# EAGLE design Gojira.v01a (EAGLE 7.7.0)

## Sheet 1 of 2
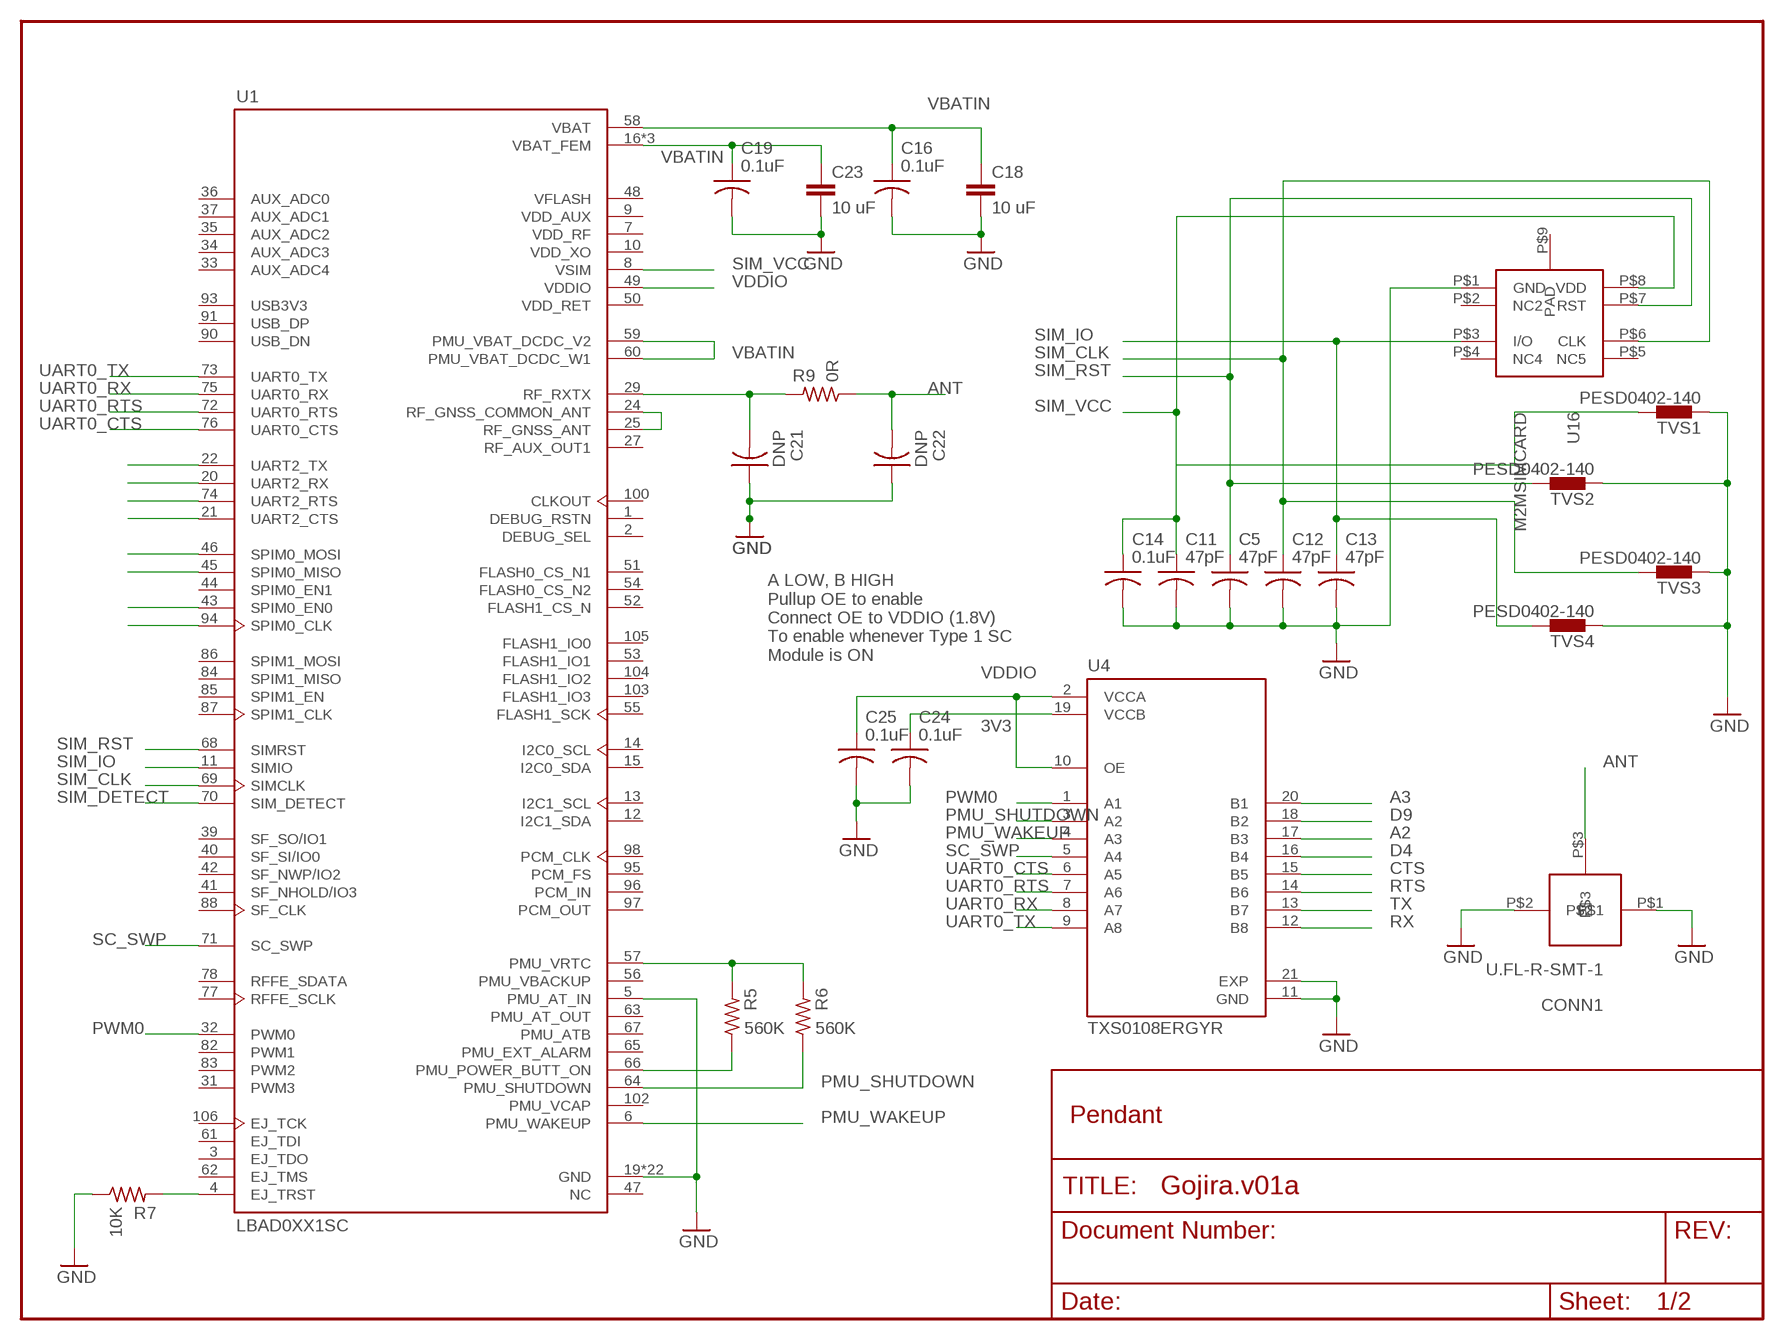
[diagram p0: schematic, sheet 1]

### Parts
C5  47pF  C-US  [C0402_B]
C11  47pF  C-US  [C0402_B]
C12  47pF  C-US  [C0402_B]
C13  47pF  C-US  [C0402_B]
C14  0.1uF  C-US  [C0402_B]
C16  0.1uF  C-US  [C0402_B]
C18  10 uF  CAP0603-CAP  [0603-CAP]
C19  0.1uF  C-US  [C0402_B]
C21  DNP  C-US  [C0402_B]
C22  DNP  C-US  [C0402_B]
C23  10 uF  CAP0603-CAP  [0603-CAP]
C24  0.1uF  C-US  [C0402_B]
C25  0.1uF  C-US  [C0402_B]
CONN1  U.FL-R-SMT-1  [U.FL-R-SMT-1]
R5  560K  R-US_  [R0402_B]
R6  560K  R-US_  [R0402_B]
R7  10K  R-US_  [R0402_B]
R9  0R  R-US_  [R0402_B]
TVS1  PESD0402-140  BLM15H  [0402]
TVS2  PESD0402-140  BLM15H  [0402]
TVS3  PESD0402-140  BLM15H  [0402]
TVS4  PESD0402-140  BLM15H  [0402]
U1  LBAD0XX1SC  [XCVR_LBAD0XX1SC]
U4  TXS0108ERGYR  [IC_TXS0108ERGYR]
U16  M2MSIMCARD  [M2MSIMCARD]

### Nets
3V3: C24.1 U4.19(VCCB) ; also sheet 2
A2: U4.17(B3) ; also sheet 2
A3: U4.20(B1) ; also sheet 2
ANT: C22.2 CONN1.P$3 R9.1
CTS: U4.15(B5) ; also sheet 2
D4: U4.16(B4) ; also sheet 2
D9: U4.18(B2) ; also sheet 2
GND: C5.2 C11.2 C12.2 C13.2 C14.2 C16.2 C18.2 C19.2 C21.1 C22.1 C23.2 C24.2 C25.2 CONN1.P$1 CONN1.P$2 R7.1 TVS1.1 TVS2.1 TVS3.1 TVS4.1 U1.5(PMU_AT_IN) U1.19(GND) U1.23(GND) U1.26(GND) U1.28(GND) U1.30(GND) U1.38(GND) U1.79(GND) U1.80(GND) U1.81(GND) U1.89(GND) U1.92(GND) U1.99(GND) U1.101(GND) U1.107(GND) U1.108(GND) U1.109(GND) U1.110(GND) U1.111(GND) U1.112(GND) U1.113(GND) U1.114(GND) U1.115(GND) U4.11(GND) U4.21(EXP) U16.P$1(GND) ; also sheet 2
N$3: R5.2 R6.2 U1.57(PMU_VRTC)
N$5: R5.1 U1.66(PMU_POWER_BUTT_ON)
N$9: U1.24(RF_GNSS_COMMON_ANT) U1.25(RF_GNSS_ANT)
N$10: R7.2 U1.4(EJ_TRST)
N$13: U1.20(UART2_RX)
N$14: U1.22(UART2_TX)
N$16: U1.21(UART2_CTS)
N$17: U1.74(UART2_RTS)
N$18: U1.43(SPIM0_EN0)
N$19: U1.45(SPIM0_MISO)
N$20: U1.46(SPIM0_MOSI)
N$21: U1.94(SPIM0_CLK)
PMU_SHUTDOWN: R6.1 U1.64(PMU_SHUTDOWN) U4.3(A2)
PMU_WAKEUP: U1.6(PMU_WAKEUP) U4.4(A3)
PWM0: U1.32(PWM0) U4.1(A1)
RF_OUT: C21.2 R9.2 U1.29(RF_RXTX)
RTS: U4.14(B6) ; also sheet 2
RX: U4.12(B8) ; also sheet 2
SC_SWP: U1.71(SC_SWP) U4.5(A4)
SIM_CLK: C12.1 TVS3.2 U1.69(SIMCLK) U16.P$6(CLK)
SIM_DETECT: U1.70(SIM_DETECT)
SIM_IO: C13.1 TVS4.2 U1.11(SIMIO) U16.P$3(I/O)
SIM_RST: C5.1 TVS2.2 U1.68(SIMRST) U16.P$7(RST)
SIM_VCC: C11.1 C14.1 TVS1.2 U1.8(VSIM) U16.P$8(VDD)
TX: U4.13(B7) ; also sheet 2
UART0_CTS: U1.76(UART0_CTS) U4.6(A5)
UART0_RTS: U1.72(UART0_RTS) U4.7(A6)
UART0_RX: U1.75(UART0_RX) U4.8(A7)
UART0_TX: U1.73(UART0_TX) U4.9(A8)
VBATIN: C16.1 C18.1 C19.1 C23.1 U1.16(VBAT_FEM) U1.17(VBAT_FEM) U1.18(VBAT_FEM) U1.58(VBAT) U1.59(PMU_VBAT_DCDC_V2) U1.60(PMU_VBAT_DCDC_W1) ; also sheet 2
VDDIO: C25.1 U1.49(VDDIO) U4.2(VCCA) U4.10(OE)
Unconnected: U1.1(DEBUG_RSTN) U1.2(DEBUG_SEL) U1.3(EJ_TDO) U1.7(VDD_RF) U1.9(VDD_AUX) U1.10(VDD_XO) U1.12(I2C1_SDA) U1.13(I2C1_SCL) U1.14(I2C0_SCL) U1.15(I2C0_SDA) U1.27(RF_AUX_OUT1) U1.31(PWM3) U1.33(AUX_ADC4) U1.34(AUX_ADC3) U1.35(AUX_ADC2) U1.36(AUX_ADC0) U1.37(AUX_ADC1) U1.39(SF_SO/IO1) U1.40(SF_SI/IO0) U1.41(SF_NHOLD/IO3) U1.42(SF_NWP/IO2) U1.44(SPIM0_EN1) U1.47(NC) U1.48(VFLASH) U1.50(VDD_RET) U1.51(FLASH0_CS_N1) U1.52(FLASH1_CS_N) U1.53(FLASH1_IO1) U1.54(FLASH0_CS_N2) U1.55(FLASH1_SCK) U1.56(PMU_VBACKUP) U1.61(EJ_TDI) U1.62(EJ_TMS) U1.63(PMU_AT_OUT) U1.65(PMU_EXT_ALARM) U1.67(PMU_ATB) U1.77(RFFE_SCLK) U1.78(RFFE_SDATA) U1.82(PWM1) U1.83(PWM2) U1.84(SPIM1_MISO) U1.85(SPIM1_EN) U1.86(SPIM1_MOSI) U1.87(SPIM1_CLK) U1.88(SF_CLK) U1.90(USB_DN) U1.91(USB_DP) U1.93(USB3V3) U1.95(PCM_FS) U1.96(PCM_IN) U1.97(PCM_OUT) U1.98(PCM_CLK) U1.100(CLKOUT) U1.102(PMU_VCAP) U1.103(FLASH1_IO3) U1.104(FLASH1_IO2) U1.105(FLASH1_IO0) U1.106(EJ_TCK) U16.P$2(NC2) U16.P$4(NC4) U16.P$5(NC5)

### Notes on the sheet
- A LOW, B HIGH
  Pullup OE to enable
  Connect OE to VDDIO (1.8V)
  To enable whenever Type 1 SC
  Module is ON
- Pendant

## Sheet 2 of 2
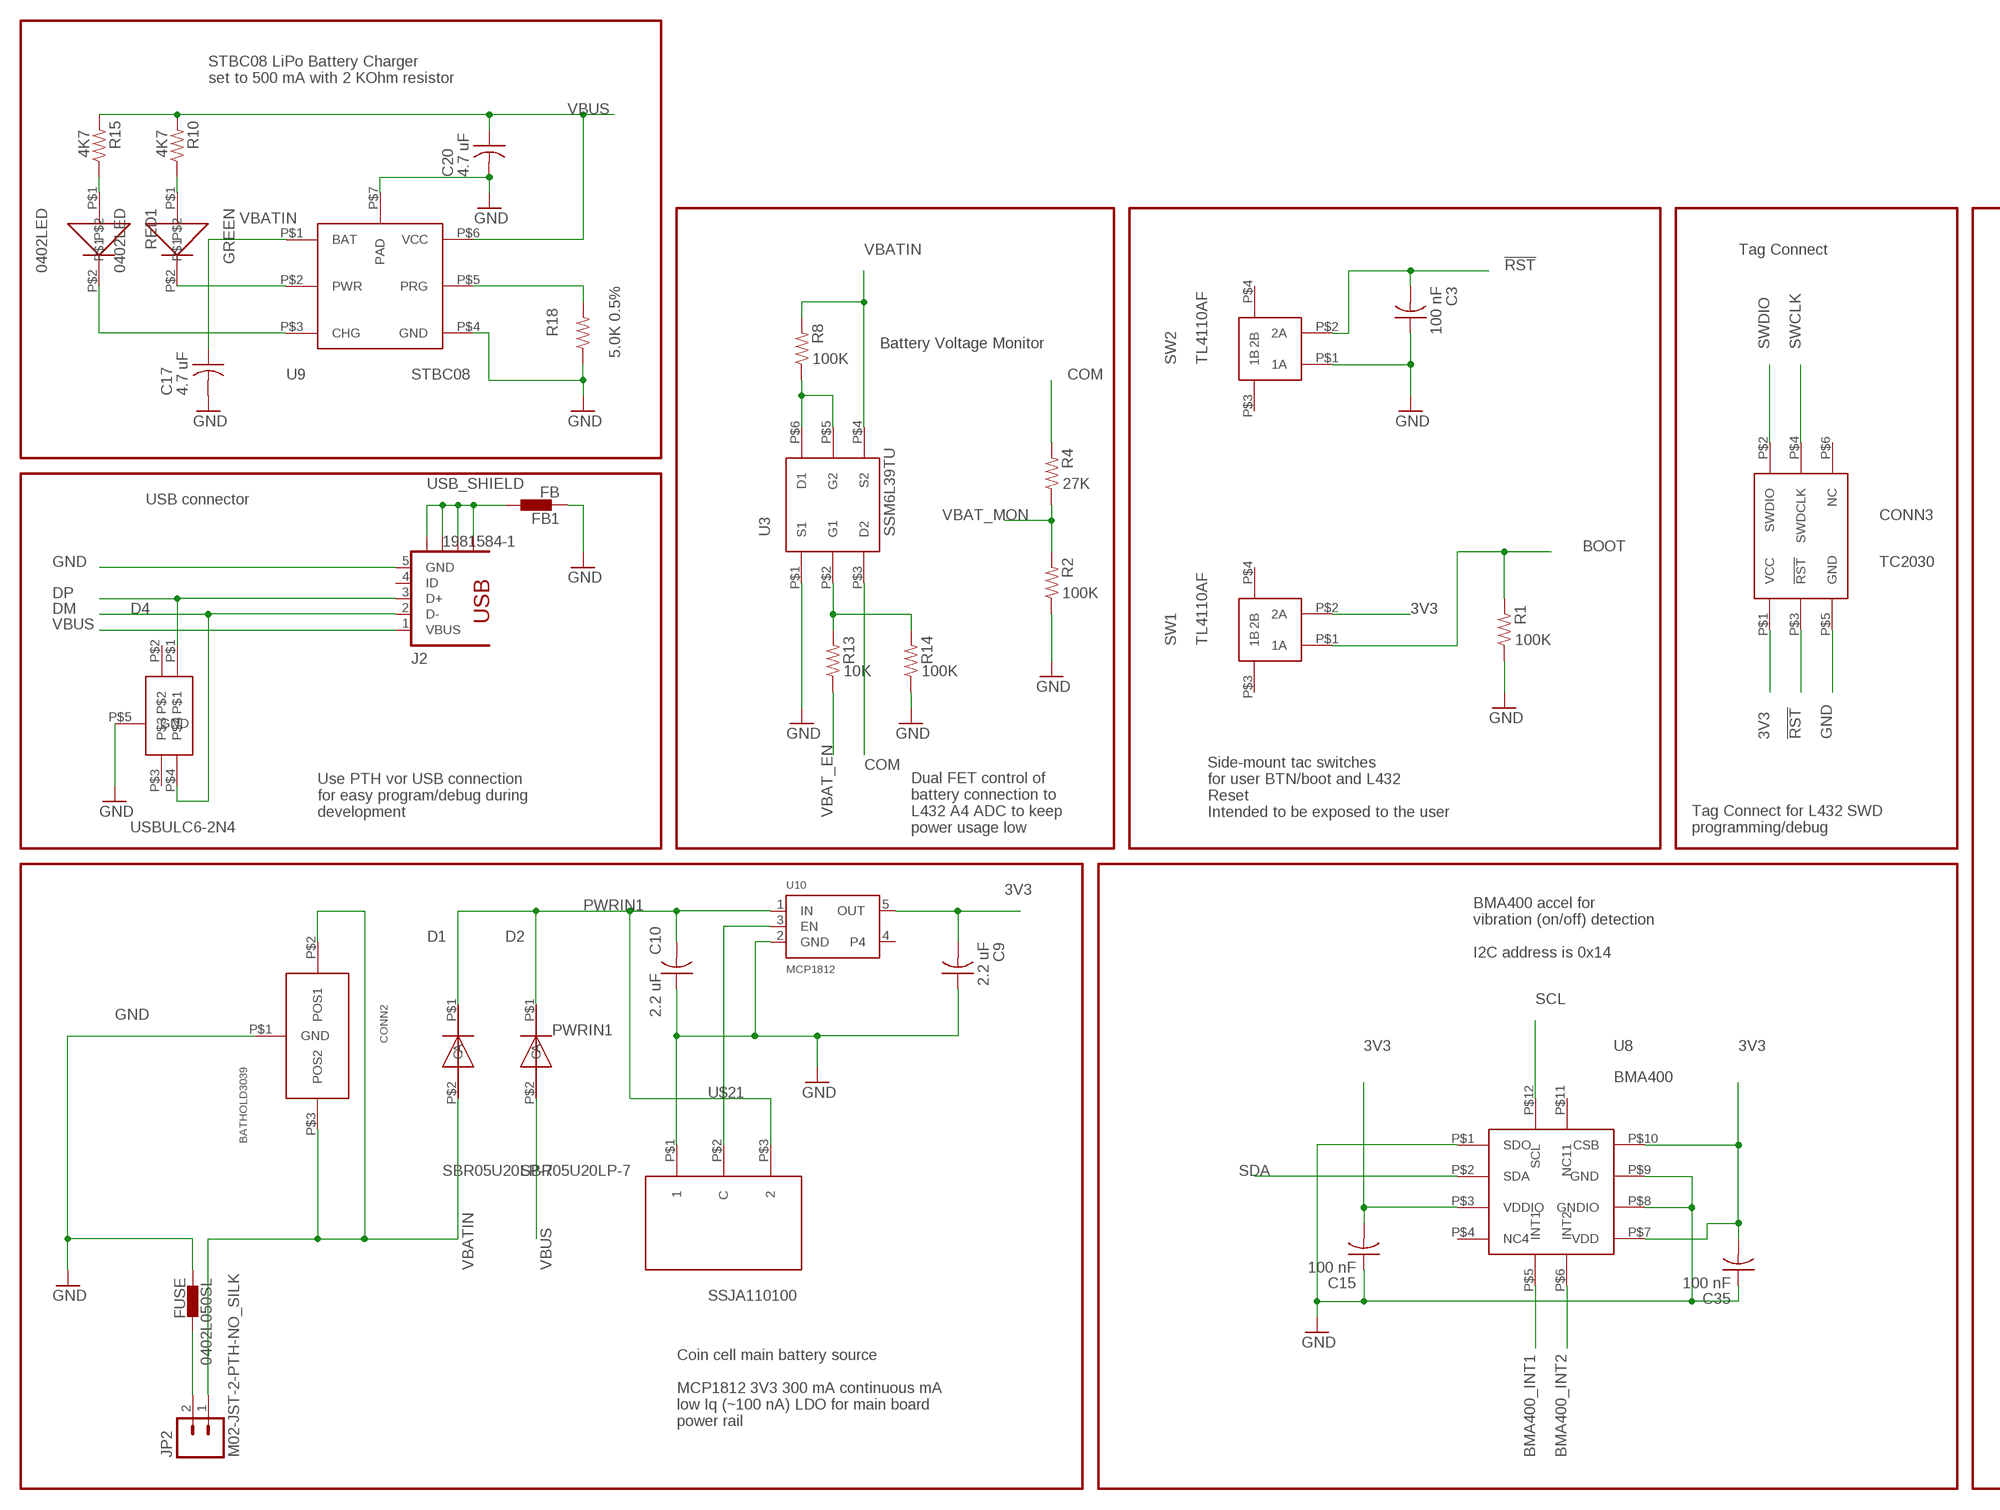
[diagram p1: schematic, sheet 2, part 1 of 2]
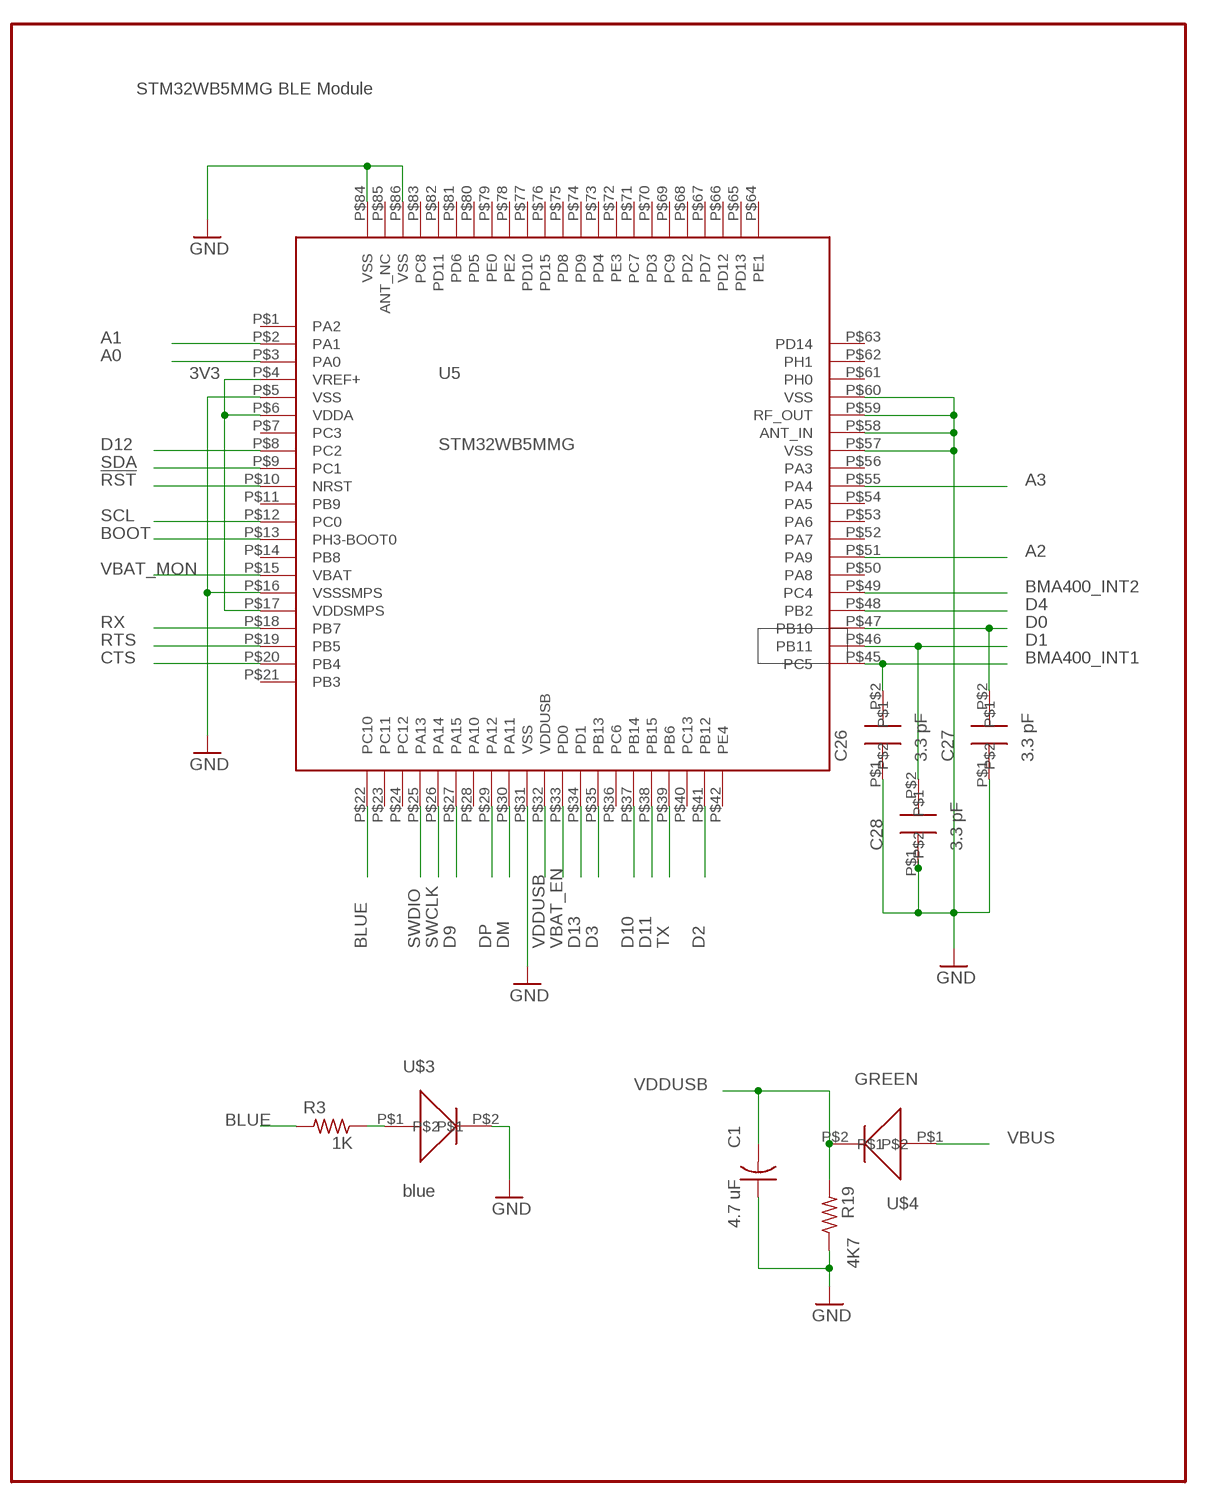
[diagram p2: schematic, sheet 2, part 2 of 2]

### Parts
0402L050SL  FUSE  BLM15H  [0402]
C1  4.7 uF  C-US  [C0402_B]
C3  100 nF  C-US  [C0402_B]
C9  2.2 uF  C-US  [C0402_B]
C10  2.2 uF  C-US  [C0402_B]
C15  100 nF  C-US  [C0402_B]
C17  4.7 uF  C-US  [C0402_B]
C20  4.7 uF  C-US  [C0402_B]
C26  3.3 pF  201CAP  [0201CAP]
C27  3.3 pF  201CAP  [0201CAP]
C28  3.3 pF  201CAP  [0201CAP]
C35  100 nF  C-US  [C0402_B]
CONN2  BATHOLD3039  [BATHOLD3039]
CONN3  TC2030  [TC2030]
D1  SBR05U20LP-7  CDSQR4148-HF  [CDSQR4148-HF]
D2  SBR05U20LP-7  CDSQR4148-HF  [CDSQR4148-HF]
D4  USBULC6-2N4  [USBULC6-2N4]
FB1  FB  BLM15H  [0402]
GREEN  0402LED  [0402LED]
J2  1981584-1  [1981584-1]
JP2  M02-JST-2-PTH-NO_SILK  [JST-2-PTH-NS]
R1  100K  R-US_  [R0402_B]
R2  100K  R-US_  [R0402_B]
R3  1K  R-US_  [R0402_B]
R4  27K  R-US_  [R0402_B]
R8  100K  R-US_  [R0402_B]
R10  4K7  R-US_  [R0402_B]
R13  10K  R-US_  [R0402_B]
R14  100K  R-US_  [R0402_B]
R15  4K7  R-US_  [R0402_B]
R18  5.0K 0.5%  R-US_  [R0402_B]
R19  4K7  R-US_  [R0402_B]
RED1  0402LED  [0402LED]
SW1  TL4110AF  [TL4110AF]
SW2  TL4110AF  [TL4110AF]
U3  SSM6L39TU  [SSM6L39TU]
U5  STM32WB5MMG  [STM32WB5MMG]
U8  BMA400  [BMA400]
U9  STBC08  [STBC08]
U10  MCP1812  VREG_SOT23-5  [SOT23-5]
U$3  blue  0402LED  [0402LED]
U$4  GREEN  0402LED  [0402LED]
U$21  SSJA110100  [SSAJ110100]

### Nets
3V3: C9.2 C15.2 C35.2 CONN3.P$1(VCC) SW1.P$2(2A) U5.P$4(VREF+) U5.P$6(VDDA) U5.P$17(VDDSMPS) U8.P$3(VDDIO) U8.P$7(VDD) U8.P$10(CSB) U10.5(OUT) ; also sheet 1
!RST: C3.2 CONN3.P$3(!RST) SW2.P$2(2A) U5.P$10(NRST)
A0: U5.P$3(PA0)
A1: U5.P$2(PA1)
A2: U5.P$51(PA9) ; also sheet 1
A3: U5.P$55(PA4) ; also sheet 1
BLUE: R3.2 U5.P$22(PC10)
BMA400_INT1: C26.P$2 U5.P$45(PC5) U8.P$5(INT1)
BMA400_INT2: U5.P$49(PC4) U8.P$6(INT2)
BOOT: R1.2 SW1.P$1(1A) U5.P$13(PH3-BOOT0)
COM: R4.2 U3.P$3(D2)
CTS: U5.P$20(PB4) ; also sheet 1
D0: C27.P$2 U5.P$47(PB10)
D1: C28.P$2 U5.P$46(PB11)
D2: U5.P$41(PB12)
D3: U5.P$35(PB13)
D4: U5.P$48(PB2) ; also sheet 1
D9: U5.P$27(PA15) ; also sheet 1
D10: U5.P$37(PB14)
D11: U5.P$38(PB15)
D12: U5.P$8(PC2)
D13: U5.P$34(PD1)
DM: D4.P$4 J2.2(D-) U5.P$30(PA11)
DP: D4.P$1 J2.3(D+) U5.P$29(PA12)
GND: 0402L050SL.1 C1.1 C3.1 C9.1 C10.1 C15.1 C17.2 C20.2 C26.P$1 C27.P$1 C28.P$1 C35.1 CONN2.P$1(GND) CONN3.P$5(GND) D4.P$5(GND) FB1.1 J2.5(GND) R1.1 R2.1 R14.1 R18.1 R19.1 SW2.P$1(1A) U3.P$1(S1) U5.P$5(VSS) U5.P$16(VSSSMPS) U5.P$31(VSS) U5.P$57(VSS) U5.P$58(ANT_IN) U5.P$59(RF_OUT) U5.P$60(VSS) U5.P$84(VSS) U5.P$86(VSS) U8.P$1(SDO) U8.P$8(GNDIO) U8.P$9(GND) U9.P$4(GND) U9.P$7(PAD) U10.2(GND) U$3.P$2 U$21.P$1 ; also sheet 1
N$1: R15.1 RED1.P$1
N$4: 0402L050SL.2 JP2.2
N$7: R13.2 R14.2 U3.P$2(G1)
N$11: R3.1 U$3.P$1
N$15: R8.1 U3.P$5(G2) U3.P$6(D1)
N$22: RED1.P$2 U9.P$3(CHG)
N$23: GREEN.P$2 U9.P$2(PWR)
N$24: GREEN.P$1 R10.1
N$25: U10.3(EN) U$21.P$2(C)
N$27: R18.2 U9.P$5(PRG)
PWRIN1: C10.2 D1.P$1(C) D2.P$1(C) U10.1(IN) U$21.P$3
RTS: U5.P$19(PB5) ; also sheet 1
RX: U5.P$18(PB7) ; also sheet 1
SCL: U5.P$12(PC0) U8.P$12(SCL)
SDA: U5.P$9(PC1) U8.P$2(SDA)
SWCLK: CONN3.P$4(SWDCLK) U5.P$26(PA14)
SWDIO: CONN3.P$2(SWDIO) U5.P$25(PA13)
TX: U5.P$39(PB6) ; also sheet 1
USB_SHIELD: FB1.2 J2.S1 J2.S2 J2.S3 J2.S4
VBAT_EN: R13.1 U5.P$33(PD0)
VBAT_MON: R2.2 R4.1 U5.P$15(VBAT)
VBATIN: C17.1 CONN2.P$2(POS1) CONN2.P$3(POS2) D1.P$2(A) JP2.1 R8.2 U3.P$4(S2) U9.P$1(BAT) ; also sheet 1
VBUS: C20.1 D2.P$2(A) J2.1(VBUS) R10.2 R15.2 U9.P$6(VCC) U$4.P$1
VDDUSB: C1.2 R19.2 U5.P$32(VDDUSB) U$4.P$2
Unconnected: CONN3.P$6(NC) D4.P$2 D4.P$3 J2.4(ID) SW1.P$3(1B) SW1.P$4(2B) SW2.P$3(1B) SW2.P$4(2B) U5.P$1(PA2) U5.P$7(PC3) U5.P$11(PB9) U5.P$14(PB8) U5.P$21(PB3) U5.P$23(PC11) U5.P$24(PC12) U5.P$28(PA10) U5.P$36(PC6) U5.P$40(PC13) U5.P$42(PE4) U5.P$50(PA8) U5.P$52(PA7) U5.P$53(PA6) U5.P$54(PA5) U5.P$56(PA3) U5.P$61(PH0) U5.P$62(PH1) U5.P$63(PD14) U5.P$64(PE1) U5.P$65(PD13) U5.P$66(PD12) U5.P$67(PD7) U5.P$68(PD2) U5.P$69(PC9) U5.P$70(PD3) U5.P$71(PC7) U5.P$72(PE3) U5.P$73(PD4) U5.P$74(PD9) U5.P$75(PD8) U5.P$76(PD15) U5.P$77(PD10) U5.P$78(PE2) U5.P$79(PE0) U5.P$80(PD5) U5.P$81(PD6) U5.P$82(PD11) U5.P$83(PC8) U5.P$85(ANT_NC) U8.P$4(NC4) U8.P$11(NC11) U10.4

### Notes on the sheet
- STBC08 LiPo Battery Charger
  set to 500 mA with 2 KOhm resistor
- Tag Connect
- STM32WB5MMG BLE Module
- Battery Voltage Monitor
- USB connector
- Use PTH vor USB connection
  for easy program/debug during
  development
- Side-mount tac switches
  for user BTN/boot and L432 
  Reset
  Intended to be exposed to the user
- Dual FET control of
  battery connection to
  L432 A4 ADC to keep
  power usage low
- Tag Connect for L432 SWD 
  programming/debug
- BMA400 accel for
  vibration (on/off) detection
  
  I2C address is 0x14
- Coin cell main battery source
  
  MCP1812 3V3 300 mA continuous mA
  low Iq (~100 nA) LDO for main board 
  power rail

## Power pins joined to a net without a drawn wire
PAD: U16.P$9(PAD)

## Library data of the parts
0402L050SL FB1 TVS1-TVS4 = STM32L433SARA.AssetTracker.v01:BLM15H: EMIFIL (R) Chip Ferrite Bead for GHz Noise
C1 C3 C5 C9-C17 C19-C22 C24 C25 C35 = Spark:C-US: Capacitor
C18 C23 = SparkFun-Capacitors:CAP: Capacitor
C26-C28 = Kris:201CAP: 0201 capacitor for high-density applications (STM32WB5MMG)
CONN1 = Kris:U.FL-R-SMT-1: U.FL-R-SMT-1
CONN2 = Kris:BATHOLD3039: 2450 battery holder file:///C:/Users/kris/AppData/Local/Temp/3039.PDF
CONN3 = Kris:TC2030: TC2030 SWD pogo pin contact pad
D1 D2 = Kris:CDSQR4148-HF: ComChip's CDSQR4148-HF high speed 150 mA Io diode
D4 = Kris:USBULC6-2N4: ST TVS diode ESD Protection USBULC6-2N4
GREEN RED1 U$3 U$4 = Kris:0402LED: 0402led
J2 = con-usb:1981584-1: Receptacle, micro-USB, type A/B Tyco Electronics; MF: Hirose; MPN: ZX62-AB-5PA(11)
JP2 = SparkFun-Connectors:M02: Standard 2-pin 0.1" header. Use with
R1-R10 R13-R15 R18 R19 = Spark:R-US_: 0402 Resistor
SW1 SW2 = Kris:TL4110AF: TL4110AF side-mounted tac switch
U1 = LBAD0XX1SC:LBAD0XX1SC: LTE CAT M1 Module Check prices; AVAILABILITY: Bad; DESCRIPTION: Bluetooth Development Tools (802.15.1); MF: Murata Power Solutions; MP: LBAD0XX1SC; PACKAGE: None; PRICE: None
U3 = Kris:SSM6L39TU: SSM6L39TU Dual Mosfet https://www.mouser.com/datasheet/2/408/SSM6L39TU_datasheet_en_20140301-771389.pdf
U4 = TXS0108ERGYR:TXS0108ERGYR: 8-bit bidirectional voltage-level shifter for open-drain and push-pull application 20-VQFN -40 to 85; DESCRIPTION: 8-bit bidirectional voltage-level shifter for open-drain and push-pull application 20-VQFN -40 to 85; DIGI-KEY_PART_NUMBER: 296-24806-1-ND; MF: Texas Instruments; MP: TXS0108ERGYR; PACKAGE: VQFN-20 Texas Instruments; PURCHASE-URL: https://pricing.snapeda.com/search/part/TXS0108ERGYR/?ref=eda
U5 = Kris:STM32WB5MMG: STM32WB5MMG BLE Module
U8 = Kris:BMA400: BMA400 https://ae-bst.resource.bosch.com/media/_tech/media/datasheets/BST-BMA400-DS000-02.pdf
U9 = Kris:STBC08: STBC08
U10 = ModernDevice:VREG_SOT23-5: SOT23-5 Fixed Voltage Regulators To better organise some of the SOT23-5 fixed voltage regulators in this library, this new part was created. Part Current Out V Out V In V Dropout Digikey Part No. ADP121 150mA 3.3V 3.4-5.5V 0.09V @ 150mA ADP121-AUJZ33R7CT-ND ADP121 150mA 3.0V 3.1-5.5V 0.09V @ 150mA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
U16 = Kris:M2MSIMCARD: M2M Sim Card
U$21 = Kris:SSJA110100: ALPS SSJA110100 SPDT slide switch with lugs

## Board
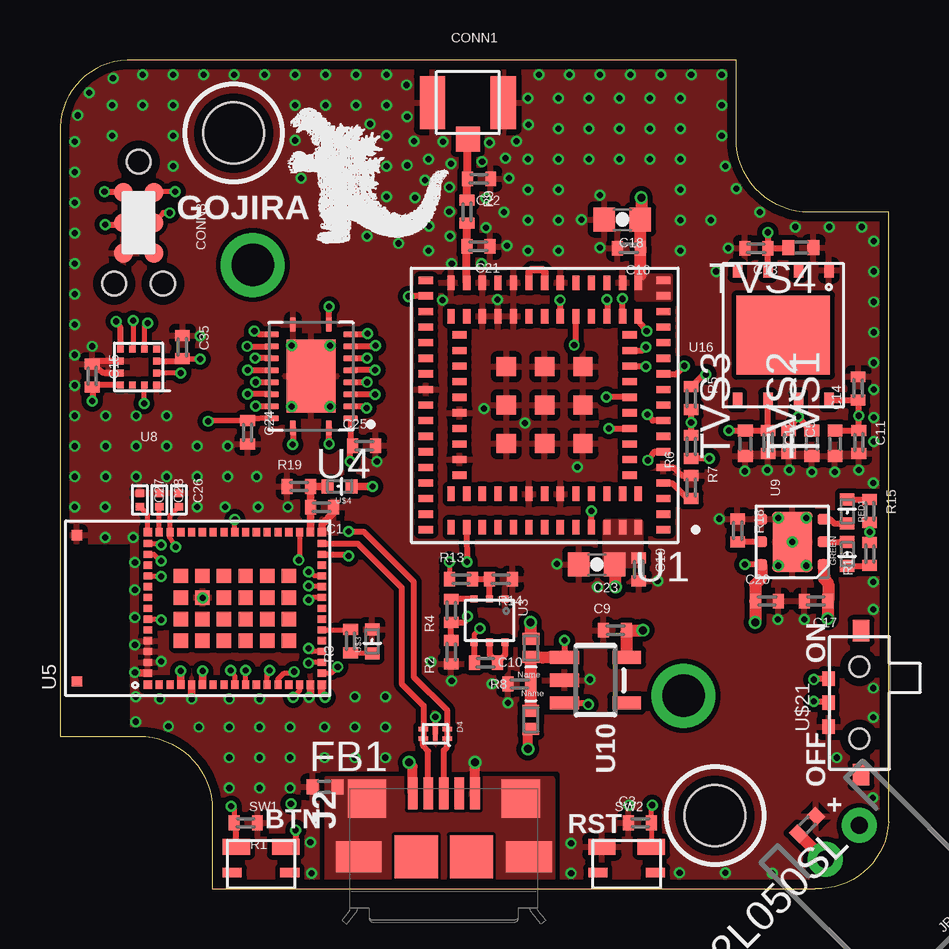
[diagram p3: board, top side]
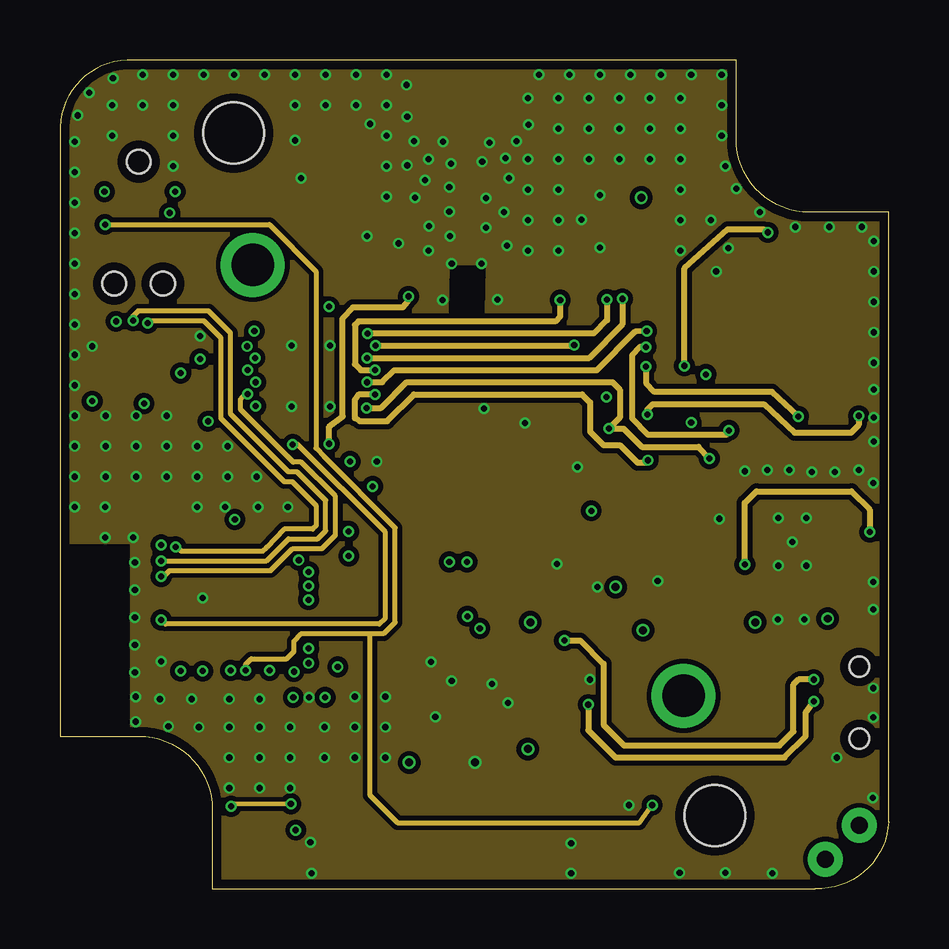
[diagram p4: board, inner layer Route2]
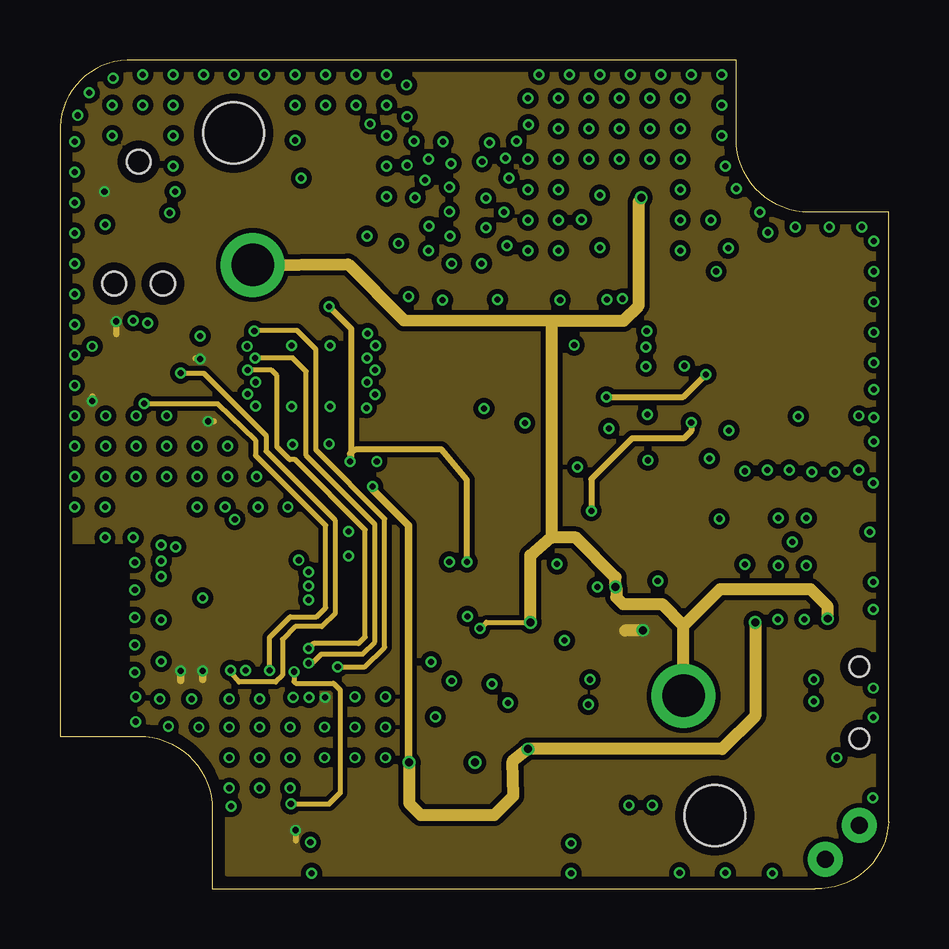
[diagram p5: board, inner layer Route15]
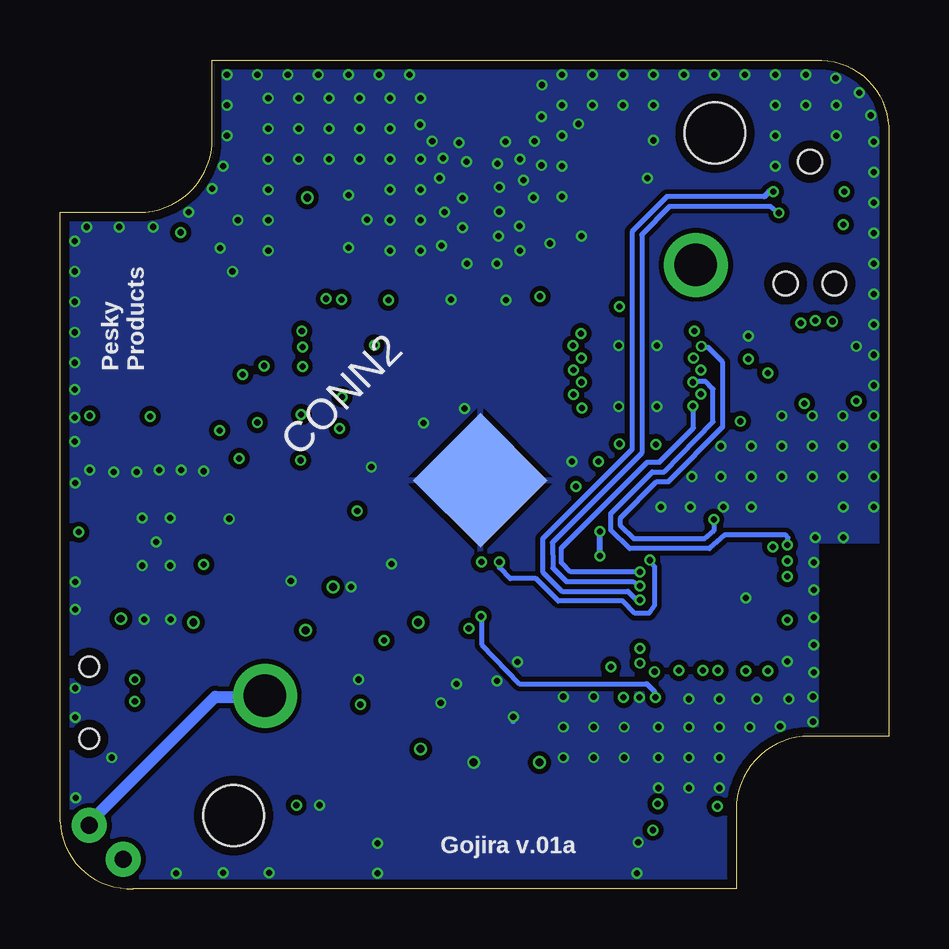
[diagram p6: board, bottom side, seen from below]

Size 34.54 x 34.54 mm. Coordinates in mm from the lower left corner, seen from the top.
Outline: 0,31.5 0,6.35 3.3,6.35 arc-90 6.35,3.3 6.35,0 31.5,0 arc90 34.54,2.79 34.54,28.19 31.24,28.19 arc-90 28.19,31.24 28.19,34.54 2.79,34.54 arc90 0,31.5
Copper layers (1*2*15*16): Top 0.035559375mm / dielectric 0.17018125mm / Route2 0.01778125mm / dielectric 47mil / Route15 0.01778125mm / dielectric 0.17018125mm / Bottom 0.035559375mm
Design rules "oshpark-4layer *": minimum track width 5mil, minimum drill 10mil, track to track 5mil, track to pad 5mil, pad to pad 5mil, via to via 5mil, smd to smd 5mil, copper to edge 15mil, drill to drill 6mil, minimum pad ring 4mil, minimum via ring 4mil, stop-mask expansion 2.5mil, vias tented up to drill 20mil, thermal gap 10mil
Holes 2.54 mm at 7.24,31.5 27.3,3.05

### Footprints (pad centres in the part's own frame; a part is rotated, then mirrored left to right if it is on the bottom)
0402 = smd 0.5 x 0.61: 1 -0.5,0; 2 0.55,0
C0402_B = smd 0.457 x 0.61: 1 -0.483,0; 2 0.483,0
0603-CAP = smd 0.9 x 1: 1 -0.75,0; 2 0.75,0
0201CAP = smd 0.32 x 0.36: P$1 -0.28,0; P$2 0.28,0
U.FL-R-SMT-1 = smd 1.05 x 2.2: P$1 -1.475,0; P$2 1.475,0 | smd 1 x 1.05: P$3 0,-1.525
BATHOLD3039 = smd 3.96 x 3.96: P$1 0,0 | drill 1.778: P$2 -12.7,0; P$3 12.7,0
TC2030 = smd 0.787 x 0.787: P$1 -1.27,-0.635; P$2 -1.27,0.635; P$3 0,-0.635; P$4 0,0.635; P$5 1.27,-0.635; P$6 1.27,0.635 | hole 0.991: -2.54,0; 2.54,1.016; 2.54,-1.016
CDSQR4148-HF = smd 0.7 x 0.5: P$1 0,0.375; P$2 0,-0.375
USBULC6-2N4 = smd 0.2 x 0.4: P$1 0.2,0.5; P$2 -0.2,0.5; P$3 -0.2,-0.5; P$4 0.2,-0.5 | smd 0.6 x 0.2: P$5 0,0
0402LED = smd 0.5 x 0.6: P$1 -0.5,0; P$2 0.5,0
1981584-1 = smd 0.4 x 1.35: 1 -1.3,4.1; 2 -0.65,4.1; 3 0,4.1; 4 0.65,4.1; 5 1.3,4.1 | smd 1.8 x 1.8: M1 -1.15,1.45; M2 1.15,1.45 | smd 1.9 x 1.3: S1 -3.55,1.45; S2 3.55,1.45 | smd 1.6 x 1.6: S3 -3.2,3.885; S4 3.2,3.885
JST-2-PTH-NS = drill 0.7 pad 1.448: 1 -1,0; 2 1,0
R0402_B = smd 0.457 x 0.61: 1 -0.483,0; 2 0.483,0
TL4110AF = smd 1.14 x 0.65: P$1 -1.03,0.725; P$2 1.03,0.725 | smd 0.8 x 0.4: P$3 -1.2,-0.35; P$4 1.2,-0.35
XCVR_LBAD0XX1SC = smd 0.6 x 0.3: 1 -4.95,5.2; 2 -4.95,4.55; 3 -4.95,3.9; 4 -4.95,3.25; 5 -4.95,2.6; 6 -4.95,1.95; 7 -4.95,1.3; 8 -4.95,0.65; 9 -4.95,0; 10 -4.95,-0.65; 11 -4.95,-1.3; 12 -4.95,-1.95; 13 -4.95,-2.6; 14 -4.95,-3.25; 15 -4.95,-3.9; 16 -4.95,-4.55; 17 -4.95,-5.2; 31 4.95,-5.2; 32 4.95,-4.55; 33 4.95,-3.9; 34 4.95,-3.25; 35 4.95,-2.6; 36 4.95,-1.95; 37 4.95,-1.3; 38 4.95,-0.65; 39 4.95,0; 40 4.95,0.65; 41 4.95,1.3; 42 4.95,1.95; 43 4.95,2.6; 44 4.95,3.25; 45 4.95,3.9; 46 4.95,4.55; 47 4.95,5.2; 61 -3.55,2.925; 62 -3.55,2.275; 63 -3.55,1.625; 64 -3.55,0.975; 65 -3.55,0.325; 66 -3.55,-0.325; 67 -3.55,-0.975; 68 -3.55,-1.625; 69 -3.55,-2.275; 70 -3.55,-2.925; 84 3.55,-2.925; 85 3.55,-2.275; 86 3.55,-1.625; 87 3.55,-0.975; 88 3.55,-0.325; 89 3.55,0.325; 90 3.55,0.975; 91 3.55,1.625; 92 3.55,2.275; 93 3.55,2.925 | smd 0.3 x 0.6: 18 -3.9,-5.1; 19 -3.25,-5.1; 20 -2.6,-5.1; 21 -1.95,-5.1; 22 -1.3,-5.1; 23 -0.65,-5.1; 24 0,-5.1; 25 0.65,-5.1; 26 1.3,-5.1; 27 1.95,-5.1; 28 2.6,-5.1; 29 3.25,-5.1; 30 3.9,-5.1; 48 3.9,5.1; 49 3.25,5.1; 50 2.6,5.1; 51 1.95,5.1; 52 1.3,5.1; 53 0.65,5.1; 54 0,5.1; 55 -0.65,5.1; 56 -1.3,5.1; 57 -1.95,5.1; 58 -2.6,5.1; 59 -3.25,5.1; 60 -3.9,5.1; 71 -3.9,-3.7; 72 -3.25,-3.7; 73 -2.6,-3.7; 74 -1.95,-3.7; 75 -1.3,-3.7; 76 -0.65,-3.7; 77 0,-3.7; 78 0.65,-3.7; 79 1.3,-3.7; 80 1.95,-3.7; 81 2.6,-3.7; 82 3.25,-3.7; 83 3.9,-3.7; 94 3.9,3.7; 95 3.25,3.7; 96 2.6,3.7; 97 1.95,3.7; 98 1.3,3.7; 99 0.65,3.7; 100 0,3.7; 101 -0.65,3.7; 102 -1.3,3.7; 103 -1.95,3.7; 104 -2.6,3.7; 105 -3.25,3.7; 106 -3.9,3.7 | smd 0.8 x 0.8: 107 -1.6,1.6; 108 0,1.6; 109 1.6,1.6; 110 -1.6,0; 111 0,0; 112 1.6,0; 113 -1.6,-1.6; 114 0,-1.6; 115 1.6,-1.6
SSM6L39TU = smd 0.3 x 0.3: P$1 -0.9,0.65; P$2 -0.9,0; P$3 -0.9,-0.65; P$4 0.9,-0.65; P$5 0.9,0; P$6 0.9,0.65
IC_TXS0108ERGYR = smd 0.24 x 0.6: 1 -0.75,2.15; 10 -0.75,-2.15; 11 0.75,-2.15; 20 0.75,2.15 | smd 0.6 x 0.24: 2 -1.65,1.75; 3 -1.65,1.25; 4 -1.65,0.75; 5 -1.65,0.25; 6 -1.65,-0.25; 7 -1.65,-0.75; 8 -1.65,-1.25; 9 -1.65,-1.75; 12 1.65,-1.75; 13 1.65,-1.25; 14 1.65,-0.75; 15 1.65,-0.25; 16 1.65,0.25; 17 1.65,0.75; 18 1.65,1.25; 19 1.65,1.75 | smd 2.05 x 3.05: 21 0,0
STM32WB5MMG = smd 0.35 x 0.35: P$1 -3.175,2.075; P$17 -3.175,-5.175; P$31 3.175,-5.175; P$47 3.175,2.075 | smd 0.35 x 0.3: P$2 -3.175,1.6; P$3 -3.175,1.15; P$4 -3.175,0.7; P$5 -3.175,0.25; P$6 -3.175,-0.2; P$7 -3.175,-0.65; P$8 -3.175,-1.1; P$9 -3.175,-1.55; P$10 -3.175,-2; P$11 -3.175,-2.45; P$12 -3.175,-2.9; P$13 -3.175,-3.35; P$14 -3.175,-3.8; P$15 -3.175,-4.25; P$16 -3.175,-4.7; P$32 3.175,-4.7; P$33 3.175,-4.25; P$34 3.175,-3.8; P$35 3.175,-3.35; P$36 3.175,-2.9; P$37 3.175,-2.45; P$38 3.175,-2; P$39 3.175,-1.55; P$40 3.175,-1.1; P$41 3.175,-0.65; P$42 3.175,-0.2; P$43 3.175,0.25; P$44 3.175,0.7; P$45 3.175,1.15; P$46 3.175,1.6 | smd 0.3 x 0.35: P$18 -2.7,-5.175; P$19 -2.25,-5.175; P$20 -1.8,-5.175; P$21 -1.35,-5.175; P$22 -0.9,-5.175; P$23 -0.45,-5.175; P$24 0,-5.175; P$25 0.45,-5.175; P$26 0.9,-5.175; P$27 1.35,-5.175; P$28 1.8,-5.175; P$29 2.25,-5.175; P$30 2.7,-5.175; P$48 2.7,2.075; P$49 2.25,2.075; P$50 1.8,2.075; P$51 1.35,2.075; P$52 0.9,2.075; P$53 0.45,2.075; P$54 0,2.075; P$55 -0.45,2.075; P$56 -0.9,2.075; P$57 -1.35,2.075; P$58 -1.8,2.075; P$59 -2.25,2.075; P$60 -2.7,2.075 | smd 0.6 x 0.6: P$61 -1.35,0.7; P$62 -1.35,-0.2; P$63 -1.35,-1.1; P$64 -1.35,-2; P$65 -1.35,-2.9; P$66 -1.35,-3.8; P$67 -0.45,-3.8; P$68 0.45,-3.8; P$69 1.35,-3.8; P$70 1.35,-2.9; P$71 1.35,-2; P$72 1.35,-1.1; P$73 1.35,-0.2; P$74 1.35,0.7; P$75 0.45,0.7; P$76 -0.45,0.7; P$77 -0.45,-0.2; P$78 -0.45,-1.1; P$79 -0.45,-2; P$80 -0.45,-2.9; P$81 0.45,-2.9; P$82 0.45,-2; P$83 0.45,-1.1; P$84 0.45,-0.2 | smd 0.43 x 0.43: P$85 -3.05,5.035; P$86 3.05,5.035
BMA400 = smd 0.29 x 0.28: P$1 -0.755,0.75; P$2 -0.755,0.25; P$3 -0.755,-0.25; P$4 -0.755,-0.75; P$7 0.755,-0.75; P$8 0.755,-0.25; P$9 0.755,0.25; P$10 0.755,0.75 | smd 0.28 x 0.29: P$5 -0.25,-0.75; P$6 0.25,-0.75; P$11 0.25,0.75; P$12 -0.25,0.75
STBC08 = smd 0.45 x 0.5: P$1 -0.95,-1.3; P$2 0,-1.3; P$3 0.95,-1.3; P$4 0.95,1.3; P$5 0,1.3; P$6 -0.95,1.3 | smd 2.5 x 1.69: P$7 0,0
SOT23-5 = smd 0.55 x 1.2: 1 -0.95,-1.3; 2 0,-1.3; 3 0.95,-1.3; 4 0.95,1.3; 5 -0.95,1.3
M2MSIMCARD = smd 0.4 x 0.6: P$1 -1.905,-2.7; P$2 -0.635,-2.7; P$3 0.635,-2.7; P$4 1.905,-2.7; P$5 1.905,2.7; P$6 0.635,2.7; P$7 -0.635,2.7; P$8 -1.905,2.7 | smd 3.9 x 3.3: P$9 0,0
SSAJ110100 = smd 0.6 x 0.51: P$1 -1,1.28; P$2 0,1.285; P$3 1,1.285 | smd 0.9 x 0.7: P$4 3,-0.07; P$5 -3,-0.07 | hole 0.83: -1.5,0; 1.5,0

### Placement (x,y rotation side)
0402L050SL  31.17,2.67 225 top
C1  10.92,15.9 180 top
C3  24.18,2.74 0 top
C5  30.38,18.62 270 top
C9  23.14,10.77 0 top
C10  19.15,8.53 0 top
C11  33.3,18.62 270 top
C12  29.51,18.62 270 top
C13  29.03,26.7 180 top
C14  33.27,20.85 90 top
C15  1.35,21.39 270 top
C16  23.72,26.7 180 top
C17  31.52,11.99 180 top
C18  23.44,27.89 180 top
C19  24.13,13.31 270 top
C20  29.46,11.99 0 top
C21  17.45,26.77 180 top
C22  17.48,29.59 180 top
C23  22.38,13.51 180 top
C24  7.82,19.02 270 top
C25  12.67,18.47 0 top
C26  4.95,16.21 270 top
C27  3.33,16.21 270 top
C28  4.14,16.21 270 top
C35  5.11,22.58 270 top
CONN1  17.01,32.77 0 top
CONN2  17.02,17.02 45 bottom
CONN3  3.28,27.76 270 top
D1  19.63,10.03 180 top
D2  19.63,7.04 0 top
D4  15.65,6.45 270 top
FB1  11.02,4.24 0 top
GREEN  32.82,13.94 90 top
J2  16,-0.13 0 top
JP2  32.61,1.93 225 top
R1  7.75,2.74 180 top
R2  16.31,9.86 90 top
R3  12.12,10.31 90 top
R4  16.31,11.58 90 top
R5  26.31,20.45 270 top
R6  26.31,18.41 90 top
R7  26.31,16.74 270 top
R8  17.75,9.42 180 top
R9  16.97,28.22 270 top
R10  33.76,13.94 90 top
R13  16.71,12.9 0 top
R14  18.39,12.9 180 top
R15  33.76,15.75 270 top
R18  28.24,14.94 270 top
R19  9.96,16.76 0 top
RED1  32.82,15.72 270 top
SW1  8.38,1.02 0 top
SW2  23.62,1.02 0 top
TVS1  32.31,18.54 90 top
TVS2  31.34,18.54 90 top
TVS3  28.57,18.54 90 top
TVS4  30.91,26.72 180 top
U1  20.21,20.16 180 top
U3  17.91,11.18 270 top
U4  10.46,21.36 180 top
U5  5.74,11.68 90 top
U8  3.28,21.74 180 top
U9  30.53,14.45 90 top
U10  22.33,8.69 270 top
U16  30.15,23.07 180 top
U$3  13.02,10.31 90 top
U$4  11.66,16.76 180 top
U$21  33.32,7.75 90 top

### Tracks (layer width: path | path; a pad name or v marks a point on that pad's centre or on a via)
3V3  (via drill 0.25, 0.33)
  Top 0.254: 9.64,1.74 SW1.P$2 9.83,1.96 v9.83,2.44 | 1.36,20.99 1.36,20.46 v1.35,20.32 | U8.P$10 1.36,20.99 | 1.36,20.99 C15.2 | v5.84,22.07 C35.2 5.1,21.99 U8.P$3 | U8.P$7 2.52,23.39 v2.34,23.65 | v6.17,19.48 C24.1 7.85,19.58 U4.19 | CONN3.P$1 1.93,29.03 v1.85,29.06
  Top 0.305: U5.P$17 10.91,8.11 v11.05,7.98 | U5.P$4 5.04,8.6 v5.03,9.07 | U5.P$6 5.94,8.66 v5.94,9.07
  Top 0.508: v24.31,10.77 C9.2 23.63,10.51 U10.5
  Route15 0.254: v9.83,2.44 9.83,2.01 | v1.35,20.32 1.35,20.52 | v5.84,22.07 5.64,22.1 | v2.34,23.65 2.34,23.14 2.36,23.11 | v6.17,19.48 6.43,19.48 | v1.85,29.06 1.88,29.03
  Route15 0.305: v11.05,7.98 11,8.03 | v5.03,9.07 5.03,8.69 | v5.94,9.07 5.94,8.71
  Route15 0.508: v24.31,10.77 23.6,10.77 23.57,10.74
  pour Route15 (isolate 0.203): 6.99,0.64 31.45,0.64 arc90 33.91,2.79 33.91,27.56 31.24,27.56 arc-90 27.56,31.24 27.56,33.91 2.79,33.91 arc90 0.64,31.5 0.64,6.99 3.3,6.99 arc-90 6.99,3.3
!RST  (via drill 0.25)
  Top 0.203: U5.P$10 v7.74,9.09 v7.75,9.09 | v24.69,3.48 24.66,3.45 C3.2 24.66,1.75 SW2.P$2
  Top 0.254: v1.88,27.69 2.56,27.69 CONN3.P$3
  Route2 0.203: v24.69,3.48 24.66,3.45 24.16,2.74 14.07,2.74 12.93,3.89 12.93,10.57 12.98,10.62 | v1.88,27.69 8.74,27.69 10.67,25.73 10.67,18.36 11.02,17.98 13.97,15.04 13.97,11.1 13.49,10.62 12.98,10.62 | 12.98,10.62 10.06,10.62 9.75,10.31 9.75,9.88 9.45,9.58 7.98,9.58 7.75,9.35 v7.75,9.09
A2  (via drill 0.25)
  Top 0.203: U5.P$51 4.09,13.03 v4.22,13.01
  Top 0.254: U4.17 7.86,20.61 v7.82,20.62
  Route2 0.203: v7.82,20.62 7.7,20.62 7.52,20.4 7.52,19.99 9.73,17.78 10.06,17.78 11.48,16.36 11.48,14.73 10.92,14.17 9.7,14.17 8.79,13.26 4.57,13.26 4.32,13.01 v4.22,13.01
A3  (via drill 0.25)
  Top 0.203: U5.P$55 4.21,11.23 v4.22,11.2
  Top 0.254: U4.20 9.71,18.63 v9.7,18.52
  Route2 0.203: v9.7,18.52 9.91,18.52 13.56,14.86 13.56,11.28 13.31,11.02 4.39,11.02 v4.22,11.2
ANT
  Top 0.33: R9.1 16.97,29.57 C22.2 16.99,31.23 CONN1.P$3
BLUE
  Top 0.203: U5.P$22 12.11,10.78 R3.2
BMA400_INT1  (via drill 0.25)
  Top 0.203: C26.P$2 4.59,15.54 U5.P$45 4.57,14.84 4.57,14.66 v4.83,14.25 | U8.P$5 3.53,23.44 v3.66,23.57
  Route2 0.203: v3.66,23.57 3.66,23.67 5.99,23.67 6.71,22.96 6.71,19.61 9.35,16.97 9.68,16.97 10.67,15.98 10.67,15.11 10.54,14.99 9.35,14.99 8.61,14.22 8.46,14.07 5.05,14.07 4.9,14.22 4.78,14.22 v4.83,14.25
BMA400_INT2  (via drill 0.25)
  Top 0.203: U5.P$49 3.92,13.93 v4.22,13.66 | v3.05,23.67 3.05,22.51 U8.P$6
  Route2 0.203: v4.22,13.66 8.61,13.66 9.53,14.58 10.74,14.58 11.07,14.91 11.07,16.18 9.88,17.37 9.53,17.37 7.11,19.79 7.11,23.16 6.2,24.08 3.25,24.08 3.05,23.88 v3.05,23.67
BOOT  (via drill 0.25)
  Top 0.203: R1.2 7.26,3.38 v7.14,3.43 | U5.P$13 9.09,8.73 9.35,8.99 9.7,8.99 v9.75,9.04
  Top 0.254: SW1.P$1 7.35,2.7 R1.2
  Route2 0.203: v9.63,3.53 7.11,3.5 v7.14,3.43
  Route15 0.203: v9.75,9.04 9.75,8.64 9.83,8.56 11.4,8.56 11.68,8.28 11.68,3.99 11.23,3.53 v9.63,3.53
COM
  Top 0.254: U3.P$3 16.32,12.08 R4.2
CTS  (via drill 0.25)
  Top 0.203: U5.P$20 10.51,9.88 v10.36,10.01
  Top 0.254: v7.82,21.61 8.79,21.61 U4.15
  Route15 0.203: v7.82,21.61 v7.83,21.61 U4.15 9.04,21.38 9.04,18.41 9.58,17.88 9.8,17.88 12.72,14.96 12.72,10.49 12.45,10.21 10.57,10.21 v10.36,10.01
D0
  Top 0.203: U5.P$47 3.67,15.59 C27.P$2
D1
  Top 0.203: U5.P$46 C28.P$2 | C28.P$2
D4  (via drill 0.25)
  Top 0.203: U5.P$48 4.11,14.38 v4.22,14.33
  Top 0.254: v8.15,21.11 U4.16
  Bottom 0.203: v4.22,14.33 4.19,14.63 4.29,14.73 6.83,14.73 7.47,14.17 10.79,14.17 11.58,14.94 11.58,15.65 9.86,17.37 9.35,17.37 7.32,19.46 7.32,20.83 7.62,21.13 8.13,21.13 v8.15,21.11
D9  (via drill 0.25)
  Top 0.203: U5.P$27 10.61,13.03 v10.36,13.21
  Top 0.254: v8.15,20.12 U4.18
  Bottom 0.203: v8.15,20.12 8.13,20.09 8.13,19.2 9.55,17.78 10.06,17.78 13.64,14.2 13.64,13.59 13.26,13.21 v10.36,13.21
DM
  Top 0.254: U5.P$30 12.41,14.38 14.25,12.55 14.25,8.53 15.16,7.62 15.16,6.27 D4.P$4 15.14,6.24 15.14,5.94 15.35,5.73 J2.2
DP  (via drill 0.25)
  Top 0.254: J2.3 16,5.77 16.13,5.89 16.13,6.23 D4.P$1 16.15,7.42 14.76,8.81 14.76,12.78 12.65,14.88 v12.04,14.88 | U5.P$29 11.99,13.92 v12.04,13.87
  Bottom 0.254: v12.04,13.87 v12.04,14.88
GND  (via drill 0.25, 0.33)
  Top 0.254: U8.P$8 1.39,21.99 C15.1 1.8,21.49 U8.P$9 | U1.5 25.55,17.56 25.93,17.22 R7.1 | D4.P$5 v15.65,7.16
  Top 0.305: U5.P$60 3.16,8.98 v3.12,9.02 | U5.P$5 5.49,8.36 v5.49,7.9 | U5.P$16 10.44,7.95 v10.39,7.98 | U5.P$31 10.92,15.19 11.4,15.67 C1.1
  Top 0.406: J2.5 17.3,5.01 v17.3,5.26
  Bottom 0.254: v15.65,7.16 15.65,6.99
  Bottom 0.406: v17.3,5.26 17.3,5.18
  other vias: 29.95,15.44 31.11,13.46 29.95,13.46 31.11,15.44 30.53,14.45 9.65,20.09 9.65,22.63 11.25,22.63 11.25,20.09 33.91,12.78 10.49,0.64 21.31,0.64 21.31,1.88 25.83,0.66 27.74,0.66 29.69,0.64 33.88,3.78 33.91,8.36 33.91,7.14 33.91,11.63 31.04,11.23 29.92,11.23 33.91,16.92 33.93,19.63 33.3,17.45 32.31,17.37 31.34,17.37 30.4,17.45 29.49,17.45 33.93,18.64 33.93,20.8 33.93,21.92 33.93,23.19 33.93,24.46 33.93,25.73 33.93,27 33.43,27.58 32.08,27.58 30.66,27.58 29.18,28.19 28.19,29.18 27.58,33.93 27.58,32.66 27.58,31.39 27.74,30.12 26.31,33.93 25.04,33.93 23.77,33.93 22.5,33.93 21.23,33.93 19.96,33.93 13.61,33.93 12.34,33.93 11.07,33.93 9.8,33.93 8.53,33.93 7.26,33.93 5.99,33.93 4.72,33.93 3.45,33.93 2.21,33.78 1.22,33.17 0.74,32.23 0.61,31.14 0.61,29.87 0.61,28.6 0.61,27.33 0.61,26.06 0.61,24.79 0.61,23.52 0.61,22.25 0.61,20.98 0.61,19.71 0.61,18.44 0.61,17.17 0.61,15.9 14.45,33.5 14.48,32.18 14.76,31.17 15.98,31.14 17.91,31.09 19.02,31.17 19.53,31.85 19.51,32.94 16.31,30.23 16.23,29.24 16.23,28.22 16.26,27.2 16.33,26.06 17.58,26.06 18.64,26.8 17.75,27.56 17.75,28.78 18.72,29.62 17.6,30.3 18.57,30.45 15.37,30.4 15.21,29.54 14.81,28.8 15.39,27.61 15.37,26.59 18.52,28.19 22.5,28.91 21.74,27.89 22.5,26.72 22.4,12.57 24.92,12.83 20.73,13.54 13.21,17.81 5.84,23.04 1.88,15.9 20.78,32.94 22.05,32.94 23.32,32.94 24.59,32.94 25.86,32.94 20.78,31.67 22.05,31.67 23.32,31.67 24.59,31.67 25.86,31.67 25.86,30.4 24.59,30.4 23.32,30.4 22.05,30.4 20.78,30.4 19.51,30.4 19.51,29.13 20.78,29.13 20.78,27.86 19.51,27.86 19.51,26.59 20.78,26.59 25.86,29.13 25.86,27.86 25.86,26.59 27.13,27.86 13.61,32.66 13.61,31.39 13.61,30.12 13.61,28.85 14.12,26.9 12.93,31.88 12.34,32.66 11.07,32.66 14.48,30.15 10.06,29.62 9.8,31.19 9.8,32.66 4.72,32.66 3.45,32.66 2.18,32.66 2.18,31.39 4.72,31.39 4.72,30.12 10.44,1.93 27.48,15.42 28.55,17.4 27.36,25.73 27.86,26.7 19.38,19.41 17.68,20.02 21.56,17.58 18.24,24.56 15.95,24.54 12.8,27.2 5.94,12.12 1.91,19.71 3.17,19.71 4.45,19.71 1.91,18.44 3.17,18.44 4.45,18.44 4.45,17.17 3.17,17.17 1.91,17.17 5.71,18.44 6.99,18.44 5.71,17.17 6.99,17.17 8.2,17.17 8.26,15.9 6.88,15.9 5.71,15.9 1.88,14.63 3.05,14.63 12.29,8 13.56,8 11.02,6.73 12.29,6.73 13.56,6.73 13.56,5.46 12.29,5.46 11.02,5.46 7.06,6.73 8.33,6.73 9.6,6.73 7.06,5.46 8.33,5.46 9.6,5.46 9.6,4.19 8.33,4.19 7.06,4.19 3.12,10.16 3.12,11.3 3.12,12.45 3.12,13.59 9.5,15.9 3.15,8 3.15,6.96 4.52,6.76 5.79,6.73 7.06,7.9 8.33,7.9 16.33,8.66 15.47,9.45 18.01,8.53 18.67,7.75 22.1,8.71 4.17,7.9 1.35,22.61 23.72,3.48 32.38,5.46 4.22,9.47
  pour Bottom (isolate 0.203): 6.35,0 31.5,0 arc90 34.54,2.54 34.54,28.19 31.24,28.19 arc-90 28.19,31.24 28.19,34.54 2.54,34.54 arc90 0,31.5 0,6.35 3.3,6.35 arc-90 6.35,3.3
  pour Top (isolate 0.203, rank 2): 6.35,0 31.5,0 arc90 34.54,2.54 34.54,28.19 31.24,28.19 arc-90 28.19,31.24 28.19,34.54 2.54,34.54 arc90 0,31.5 0,6.35 3.3,6.35 arc-90 6.35,3.3
  pour Route2 (isolate 0.203): 6.35,0 31.45,0 arc90 34.49,2.54 34.49,28.19 31.19,28.19 arc-90 28.14,31.24 28.14,34.54 2.49,34.54 arc90 0,31.5 0,6.35 3.3,6.35 arc-90 6.35,3.3
N$1
  Top 0.254: RED1.P$1 R15.1
N$2
  cutout Top (no thermals): 18.31,34.09 18.31,31.5 15.72,31.5 15.72,34.06
N$3  (via drill 0.25)
  Top 0.254: U1.57 22.16,15.61 v22.15,15.75 | R5.2 v26.31,19.43 R6.2
  Route15 0.254: v26.31,19.43 26.31,19.07 26.01,18.77 23.85,18.77 22.15,17.07 v22.15,15.75
N$4
  Top 0.508: JP2.2 31.84,1.22 0402L050SL.2
N$5  (via drill 0.25)
  Top 0.254: U1.66 22.85,20.48 v22.78,20.5 | v26.92,21.44 26.82,21.44 R5.1
  Route15 0.254: v22.78,20.5 25.98,20.5 v26.92,21.44
N$6
  cutout Top: 0.38,14.35 2.9,14.35 2.9,6.73 0.38,6.73
  cutout Bottom: 0.38,14.35 2.9,14.35 2.9,6.73 0.38,6.73
  cutout Route2: 0.38,14.35 2.9,14.35 2.9,6.73 0.38,6.73
  cutout Route15: 0.38,14.35 2.9,14.35 2.9,6.73 0.38,6.73
N$7
  Top 0.254: U3.P$2 R14.2 R13.2
N$9
  Top 0.305: U1.25 19.56,25.7 19.66,25.81 20.12,25.81 20.22,25.7 U1.24
N$10
  Top 0.254: U1.4 25.51,16.91 26.14,16.28 R7.2
N$11
  Top 0.203: R3.1 12.95,9.83 U$3.P$1
N$12
  cutout Route2: 16.36,25.88 17.63,25.88 17.6,24.08 16.33,24.08
N$15
  Top 0.254: U3.P$6 18.56,9.74 R8.1 17.91,9.75 U3.P$5
N$22
  Top 0.254: U9.P$3 32.09,15.4 32.28,15.21 32.81,15.21 RED1.P$2
N$23
  Top 0.254: U9.P$2 32.81,14.45 GREEN.P$2
N$24
  Top 0.254: GREEN.P$1 33.74,13.45 R10.1
N$25  (via drill 0.25)
  Top 0.254: U10.3 21.96,7.74 v22.02,7.67 | v31.42,7.8 31.99,7.8 U$21.P$2
  Route2 0.254: v22.02,7.67 22.02,6.6 23.16,5.46 30.2,5.46 31.09,6.35 31.09,7.34 v31.42,7.8
N$26
  cutout Top: 2.36,21.89 2.67,21.89 2.67,21.54 2.36,21.54
N$27
  Top 0.254: U9.P$5 R18.2
PMU_SHUTDOWN  (via drill 0.25)
  Top 0.254: v27.08,17.93 R6.1 | v22.89,19.18 U1.64 | U4.3 12.6,20.11 v12.78,20.04
  Route2 0.254: 22.78,19.13 v22.89,19.18 | v22.89,19.18 23.5,19.18 24.26,18.41 26.62,18.41 v27.08,17.93 | v12.78,20.04 13.39,20.04 14.45,21.11 23.04,21.11 23.34,20.8 23.34,19.63 v22.89,19.18
PMU_WAKEUP  (via drill 0.25)
  Top 0.254: U1.6 24.94,18.21 24.79,18.21 v24.51,17.86 | v13.13,20.6 12.15,20.6 U4.4
  Route2 0.254: v13.13,20.6 13.2,20.61 12.47,20.61 12.29,20.37 12.29,19.61 12.5,19.48 13.64,19.48 14.76,20.6 21.77,20.6 22.1,20.27 22.1,19.05 22.66,18.49 23.34,18.49 24.08,17.75 24.41,17.75 v24.51,17.86
PWM0  (via drill 0.25)
  Top 0.254: U1.32 14.67,24.71 v14.53,24.69 | v11.23,18.54 11.23,19.2 U4.1
  Route2 0.254: v11.23,18.54 11.23,19.25 11.79,19.68 11.79,23.77 12.22,24.23 14.3,24.23 14.5,24.49 v14.53,24.69
PWRIN1  (via drill 0.25)
  Top 0.254: U$21.P$3 31.45,8.75 v31.42,8.71 | v21.03,10.34 U10.1
  Top 0.508: D2.P$1 19.63,8.3 C10.2 D1.P$1 20.12,9.63 20.42,9.65 21.01,9.65 U10.1
  Route2 0.254: v31.42,8.71 30.79,8.71 30.58,8.51 30.58,6.55 30,5.97 23.52,5.97 22.66,6.83 22.66,9.37 21.69,10.34 v21.03,10.34
RF_OUT
  Top 0.33: U1.29 16.96,26.76 C21.2 R9.2
RTS  (via drill 0.25)
  Top 0.203: U5.P$19 10.4,9.43 v10.36,9.4
  Top 0.254: U4.14 8.22,22.11 v8.13,22.12
  Route15 0.203: v10.36,9.4 10.52,9.4 10.9,9.78 12.62,9.78 13.13,10.29 13.13,15.19 10.26,18.06 10.26,21.57 9.7,22.12 v8.13,22.12
RX  (via drill 0.25)
  Top 0.203: U5.P$18 11.32,8.98 v11.58,9.25
  Top 0.254: v8.1,23.24 8.18,23.24 8.31,23.11 U4.12
  Route15 0.203: 8.13,23.27 9.88,23.27 10.67,22.48 10.67,18.29 13.54,15.42 13.54,10.06 12.7,9.25 v11.58,9.25
  Route15 0.254: 8.13,23.27 v8.1,23.24
SC_SWP  (via drill 0.25)
  Top 0.254: U1.71 24.1,23.68 v24.46,23.24 | U4.5 12.75,21.11 v12.8,21.11
  Route2 0.254: v24.46,23.24 23.98,23.22 22.38,21.61 13.95,21.61 13.44,21.11 v12.8,21.11
SCL  (via drill 0.25)
  Top 0.203: v3.5,20.22 3.5,20.97 U8.P$12 | U5.P$12 8.64,8.84 8.64,8.99 v8.74,9.09
  Route15 0.203: v8.74,9.09 8.74,10.46 9.6,11.33 10.69,11.33 11.07,11.71 11.07,15.14 8.15,18.06 8.15,18.69 6.58,20.22 v3.5,20.22
SDA  (via drill 0.25)
  Top 0.203: v5.03,21.49 U8.P$2 | v7.11,9.09 7.16,9.04 7.29,8.87 U5.P$9
  Route15 0.203: v5.03,21.49 5.99,21.49 8.59,18.9 8.59,18.24 11.48,15.34 11.48,11.48 10.92,10.92 9.8,10.92 9.27,10.39 9.27,8.89 8.99,8.61 7.47,8.61 7.11,8.99 v7.11,9.09
SIM_CLK  (via drill 0.25)
  Top 0.254: U1.69 24.29,22.43 v24.43,22.58 | v27.89,19.1 TVS3.2 C12.1 U16.P$6
  Route2 0.254: v24.43,22.58 24.18,22.58 23.85,22.23 23.85,19.61 24.51,18.92 27.76,18.92 27.89,19.02 v27.89,19.1
SIM_IO  (via drill 0.25)
  Top 0.254: U16.P$3 C13.1 | C13.1 30.34,26.7 TVS4.2 | U1.11 25.7,21.46 v26.04,21.79 | v29.52,27.36 C13.1
  Route2 0.254: v26.04,21.79 26.04,25.86 27.84,27.48 29.34,27.48 v29.52,27.36
SIM_RST  (via drill 0.25)
  Top 0.254: U1.68 24.37,21.78 v24.43,21.77 | v30.79,19.68 U16.P$7 | C5.1 30.38,19.15 v30.79,19.68 | TVS2.2 31.25,19.09 v30.79,19.68
  Route2 0.254: 24.38,21.69 v24.43,21.77 24.43,21.08 24.79,20.7 29.69,20.7 30.79,19.71 v30.79,19.68
SIM_VCC  (via drill 0.25)
  Top 0.254: U1.8 24.71,19.51 v24.49,19.76 | U16.P$8 C14.1 33.3,20.34 v33.3,19.71 C11.1 TVS1.2
  Route2 0.254: 33.27,19.79 v33.3,19.71 33.3,19.33 32.97,19 30.63,19 29.34,20.19 24.71,20.19 24.49,19.96 v24.49,19.76 24.56,19.68
SWCLK  (via drill 0.25)
  Top 0.203: 4.32,28.17 CONN3.P$4 | U5.P$26 10.9,12.6 10.41,12.6 v10.36,12.62
  Top 0.254: v4.57,28.17 4.32,28.17
  Bottom 0.203: v4.57,28.17 4.93,28.45 9.12,28.45 10.29,27.25 10.29,18.16 14.02,14.43 13.99,13.36 13.44,12.8 10.67,12.8 v10.36,12.62
SWDIO  (via drill 0.25)
  Top 0.203: v4.8,29.06 3.94,29.06 | U5.P$25 10.53,12.13 v10.36,12.04
  Top 0.254: 3.94,29.06 CONN3.P$2
  Bottom 0.203: 5.18,28.85 9.25,28.85 10.69,27.38 10.69,18.31 14.43,14.58 14.43,13.21 13.61,12.39 10.87,12.39 10.52,12.04 v10.36,12.04
  Bottom 0.254: v4.8,29.06 4.98,29.06 5.18,28.85
TX  (via drill 0.25)
  Top 0.203: U5.P$39 7.29,15.27 v7.29,15.39
  Top 0.254: v7.8,22.61 U4.13
  Route15 0.254: v7.8,22.61
  Bottom 0.203: v7.29,15.39 7.29,14.91 7.67,14.58 10.62,14.58 11.18,15.11 11.18,15.44 9.68,16.97 9.17,16.97 6.91,19.25 6.91,21.95 7.52,22.55 7.75,22.55 v7.8,22.61
UART0_CTS  (via drill 0.25)
  Top 0.254: U1.76 20.86,24.51 v20.85,24.54 | v13.13,21.61 U4.6
  Route2 0.254: v13.13,21.61 12.9,21.61 12.55,21.61 12.29,21.86 12.29,23.5 12.45,23.65 20.65,23.65 U1.76 v20.86,24.53 v20.85,24.54
UART0_RTS  (via drill 0.25)
  Top 0.254: U4.7 12.71,22.11 v12.8,22.12 | U1.72 23.44,23.84 v23.44,24.59
  Route2 0.254: v12.8,22.12 22.07,22.12 23.44,23.52 v23.44,24.59
UART0_RX  (via drill 0.25)
  Top 0.254: U4.8 13.14,22.61 v13.16,22.63 | v21.44,22.66 21.51,22.73 U1.75
  Route2 0.254: v13.16,22.63 21.29,22.63 v21.44,22.66
UART0_TX  (via drill 0.25)
  Top 0.254: U4.9 12.8,23.11 v12.83,23.14 | v22.81,24.56 22.85,24.56 U1.73
  Route2 0.254: v22.81,24.56 22.81,23.7 22.25,23.14 v12.83,23.14
USB_SHIELD
  pour Top (no thermals): 20.52,0 11.13,0 11.13,4.6 20.52,4.6
VBAT_EN  (via drill 0.25)
  Top 0.203: U5.P$33 9.99,13.72 v9.96,13.69 | v16.23,13.61 R13.1
  Bottom 0.203: v9.96,13.69 9.75,13.41 9.75,11.81 9.98,11.48 10.57,11.48 11.07,11.99 13.77,11.99 14.71,12.93 15.77,12.93 16.23,13.39 v16.23,13.61
VBAT_MON  (via drill 0.25)
  Top 0.203: U5.P$15 9.99,8.26 v9.73,7.98
  Top 0.254: R2.2 R4.1 16.84,11.1 16.99,11.25 v16.99,11.35
  Bottom 0.203: v16.99,11.35 16.94,11.3 16.94,10.16 15.39,8.53 10.08,8.53 9.73,8.18 v9.73,7.98
VBATIN  (via drill 0.25, 0.33)
  Top 0.203: 17.27,10.26 17.27,10.59 v17.5,10.85
  Top 0.254: R8.2 17.27,10.26 U3.P$4
  Top 0.33: U1.18 24.11,25.68 24.21,25.58
  Top 0.406: 24.21,26.57 C16.1 | 32.03,12.01 C17.1
  Top 0.508: 24.21,25.58 24.21,26.57 | 24.21,27.8 C18.1 | C16.1 24.21,27.88 C18.1 | U9.P$1 31.86,12.92 32.03,12.7 32.03,12.01 | D1.P$2 19.63,10.97 v19.61,11.1 | v23.16,12.57 23.16,13.47 C23.1 | v24.23,28.8 24.23,27.93 C18.1 | C17.1 v32,11.25
  Route15 0.203: v17.5,10.85 17.78,11.1 v19.61,11.1
  Route15 0.254: 19.63,11.07 v19.61,11.1
  Route15 0.508: 26.04,8 CONN2.P$2 26,10.96 | CONN2.P$3 12,26.02 14.33,23.7 20.52,23.67 | 20.52,23.67 23.5,23.67 24.13,24.31 24.13,28.63 v24.23,28.8 | v32,11.25 32,11.76 31.29,12.47 27.51,12.47 26,10.96 | 20.5,14.66 20.5,23.65 20.52,23.67 | 20.5,14.66 20.52,14.63 21.51,14.63 23.16,12.98 v23.16,12.57 23.19,12.55 23.19,12.14 23.47,11.86 25.09,11.86 26,10.96 | v19.61,11.1 19.61,13.89 20.5,14.66
  Bottom 0.508: JP2.1 33.32,2.75 28.07,8 26.04,8 CONN2.P$2
  pour Top (isolate 0.254, no thermals): 22.76,15.27 24.18,15.27 24.18,13.51 22.76,13.51
  pour Top (no thermals): 25.45,24.56 24.05,24.56 24.05,25.55 25.45,25.55
VBUS  (via drill 0.25, 0.33)
  Top 0.254: U9.P$6 v28.56,13.5 v28.55,13.51 | R15.2 v33.76,14.86 R10.2
  Top 0.305: v13.03,16.76 U$4.P$1
  Top 0.406: J2.1 14.7,5.08 v14.55,5.26 | v19.51,5.82 19.51,6.4 D2.P$2
  Top 0.508: U9.P$6 29.23,12.92 28.98,12.68 C20.1 v28.98,11.1
  Route2 0.254: v28.55,13.51 28.55,16.08 29.03,16.56 32.99,16.56 33.76,15.8 v33.76,14.86
  Route15 0.254: 14.53,5.31 v14.55,5.26
  Route15 0.305: 14.53,5.31 14.53,15.14 13.03,16.64 v13.03,16.76
  Route15 0.508: v14.55,5.26 14.55,3.56 15.04,3.07 18.11,3.07 18.9,3.86 18.87,5.31 v19.51,5.82 27.61,5.82 28.98,7.19 v28.98,11.1
VDDIO  (via drill 0.25)
  Top 0.254: U1.49 16.96,14.84 v16.97,13.61 | v12.09,17.8 12.09,18.34 C25.1 12.12,18.36 U4.2 | U4.10 11.21,24.25 v11.23,24.26
  Route15 0.254: v11.23,24.26 12.14,23.34 12.14,17.86 v12.09,17.8 12.09,18.14 12.34,18.31 15.9,18.31 16.97,17.04 v16.97,13.61
VDDUSB
  Top 0.305: U5.P$32 C1.2 R19.2 U$4.P$2

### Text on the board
tPlace: GOJIRA | ON | OFF | BTN | RST | +
bPlace: Pesky / Products | Gojira v.01a
tValues: DNP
